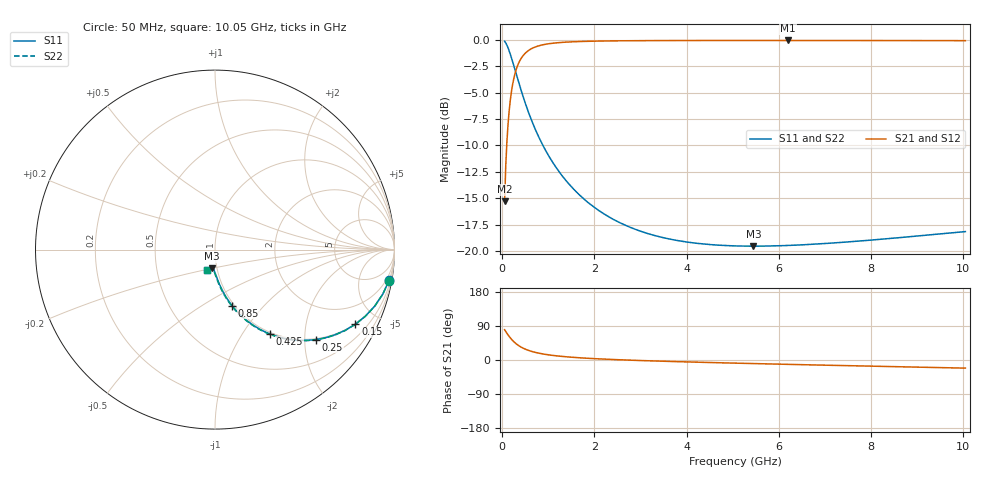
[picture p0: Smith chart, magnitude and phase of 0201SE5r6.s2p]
! AVX Thin Film Operation		Date: August 2001
! Description: Accu-P® Series, Thin Film, SMD, RF Capacitor
! Part Number: 0201ZK5R6BBW
! 50 MHz  -  10.05 GHz
! Serial Measurements
# mhz S db R 50
!	S11		S21		S12		S22
!	dB	Phase	dB	Phase	dB	Phase	dB	Phase
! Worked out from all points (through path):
!   401 points, 50 MHz to 10.05 GHz, reference 50 ohm
!   highest |S21| = -0.06 dB at 6.2 GHz (marker M1); lowest = -15.3 dB at 50 MHz (marker M2)
!   group delay of S21, straight-line fit = 13 ps
!   lowest |S11| = -19.5 dB at 5.45 GHz (marker M3), VSWR 1.24, Z = 47.5 - j10 ohm
!   |S11| at or under -10 dB: 881.3 MHz to end of sweep
!   |S22| runs from -19.6 to -0.1 dB; largest |S21 - S12| = 0
!   S11 on the Smith chart (normalised r, x): 50 MHz: 1, -11; 150 MHz: 0.98, -3.77; 250 MHz: 0.98, -2.27; 425 MHz: 0.98, -1.34; 850 MHz: 0.98, -0.68; 10.05 GHz: 0.89, -0.21
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50  -0.13 -10.0  -15.28 79.9  -15.28 79.9  -0.13 -10.1
100  -0.50 -19.5  -9.64 70.5  -9.64 70.5  -0.50 -19.6
125  -0.76 -23.9  -7.97 66.1  -7.97 66.1  -0.76 -24.0
150  -1.05 -28.0  -6.68 61.9  -6.68 61.9  -1.05 -28.1
200  -1.73 -35.4  -4.86 54.5  -4.86 54.5  -1.73 -35.5
250  -2.46 -41.7  -3.66 48.2  -3.66 48.2  -2.46 -41.8
325  -3.58 -49.3  -2.52 40.5  -2.52 40.5  -3.58 -49.5
425  -5.02 -56.9  -1.65 32.9  -1.65 32.9  -5.02 -57.2
500  -6.02 -61.2  -1.26 28.6  -1.26 28.6  -6.02 -61.5
600  -7.24 -65.7  -0.92 24.0  -0.92 24.0  -7.24 -66.1
850  -9.73 -73.1  -0.50 16.6  -0.50 16.6  -9.73 -73.6
1250  -12.60 -79.5  -0.26 10.0  -0.26 10.0  -12.60 -80.2
1725  -14.90 -83.9  -0.15 5.5  -0.15 5.5  -14.90 -84.9
2475  -17.16 -88.3  -0.09 0.9  -0.09 0.9  -17.16 -89.5
3400  -18.65 -92.0  -0.07 -3.0  -0.07 -3.0  -18.65 -93.4
4150  -19.24 -94.4  -0.06 -5.5  -0.06 -5.5  -19.24 -95.9
5050  -19.52 -97.1  -0.06 -8.3  -0.06 -8.3  -19.52 -98.6
5450  -19.55 -98.2  -0.06 -9.5  -0.06 -9.5  -19.55 -99.8
6200  -19.48 -100.2  -0.06 -11.5  -0.06 -11.5  -19.48 -101.8
6725  -19.37 -101.6  -0.06 -12.9  -0.06 -12.9  -19.37 -103.1
8400  -18.82 -106.0  -0.07 -17.3  -0.07 -17.3  -18.83 -107.3
10050  -18.17 -110.2  -0.08 -21.4  -0.08 -21.4  -18.17 -111.4
